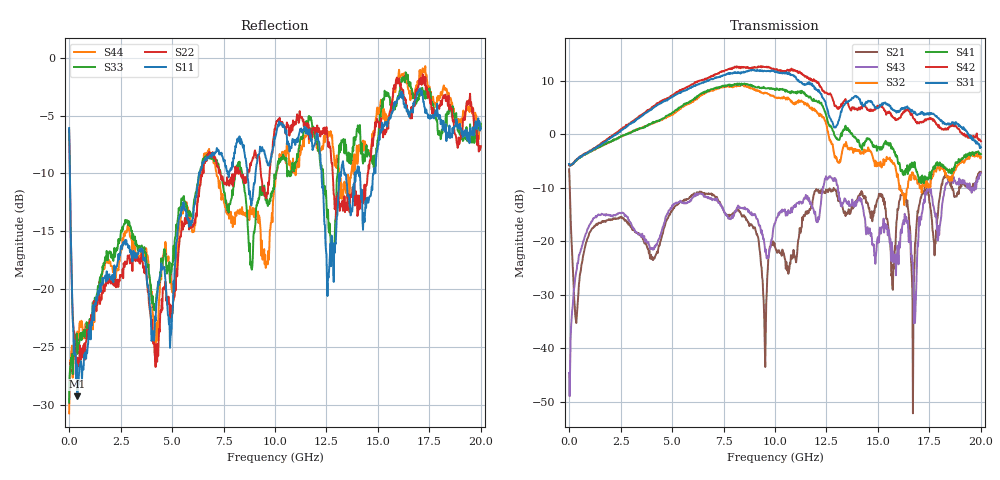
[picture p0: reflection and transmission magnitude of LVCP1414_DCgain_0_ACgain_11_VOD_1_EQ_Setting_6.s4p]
!Agilent Technologies,N5230A,MY46400459,A.07.50.48
!Agilent N5230A: A.07.50.48
!Date: Tuesday, April 17, 2012 18:31:36
!Correction: S11(Full 4 Port(1,2,3,4))
!S12(Full 4 Port(1,2,3,4))
!S13(Full 4 Port(1,2,3,4))
!S14(Full 4 Port(1,2,3,4))
!S21(Full 4 Port(1,2,3,4))
!S22(Full 4 Port(1,2,3,4))
!S23(Full 4 Port(1,2,3,4))
!S24(Full 4 Port(1,2,3,4))
!S31(Full 4 Port(1,2,3,4))
!S32(Full 4 Port(1,2,3,4))
!S33(Full 4 Port(1,2,3,4))
!S34(Full 4 Port(1,2,3,4))
!S41(Full 4 Port(1,2,3,4))
!S42(Full 4 Port(1,2,3,4))
!S43(Full 4 Port(1,2,3,4))
!S44(Full 4 Port(1,2,3,4))
!S4P File: Measurements: <S11,S12,S13,S14>,
!<S21,S22,S23,S24>,
!<S31,S32,S33,S34>,
!<S41,S42,S43,S44>:
# Hz S  dB  R 50
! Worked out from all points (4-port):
!   801 points, 300 kHz to 20 GHz, reference 50 ohm
!   strongest paths, dB at 300 kHz, 5 GHz, 10 GHz, 15 GHz, 20 GHz:
!     S31: -5.6, 7.0, 11.6, 4.9, -2.5
!     S42: -5.8, 7.3, 12.1, 5.2, -1.3
!     S41: -5.6, 4.0, 8.3, -2.4, -3.7
!     S32: -5.8, 3.7, 6.9, -5.9, -4.3
!     S43: -44.6, -13.3, -16.7, -19.2, -7.3
!     S21: -6.5, -14.2, -21.1, -12.0, -7.0
!   lowest |S11| = -29.2 dB at 400.3 MHz (marker M1), VSWR 1.07, Z = 53.3 + j1.46 ohm
!   |S11| at or under -10 dB: 37.67 MHz to 6.317 GHz (6.28 GHz wide, 198 % of centre); 12.26 GHz to 13.17 GHz (912.5 MHz wide, 7.18 % of centre); 14.13 GHz to 14.77 GHz (646.3 MHz wide, 4.47 % of centre)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
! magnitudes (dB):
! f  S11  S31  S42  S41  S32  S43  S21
! 300 kHz  -6.1  -5.6  -5.8  -5.6  -5.8  -44.6  -6.5
! 400.3 MHz  -29.2  -4.6  -4.6  -4.7  -4.7  -24.1  -32.1
! 10.1 GHz  -6.2  11.5  12.1  8.5  6.7  -15.5  -22.2
! 12.65 GHz  -17.6  3.1  7.5  1.5  -1.1  -7.9  -10.1
! 16.78 GHz  -3.8  4.2  2.7  -5.2  -8.5  -30.1  -24.8
! 17.4 GHz  -4.8  4.0  2.9  -8.2  -9.1  -10.6  -9.7
! 20 GHz  -6.1  -2.5  -1.3  -3.7  -4.3  -7.3  -7.0
